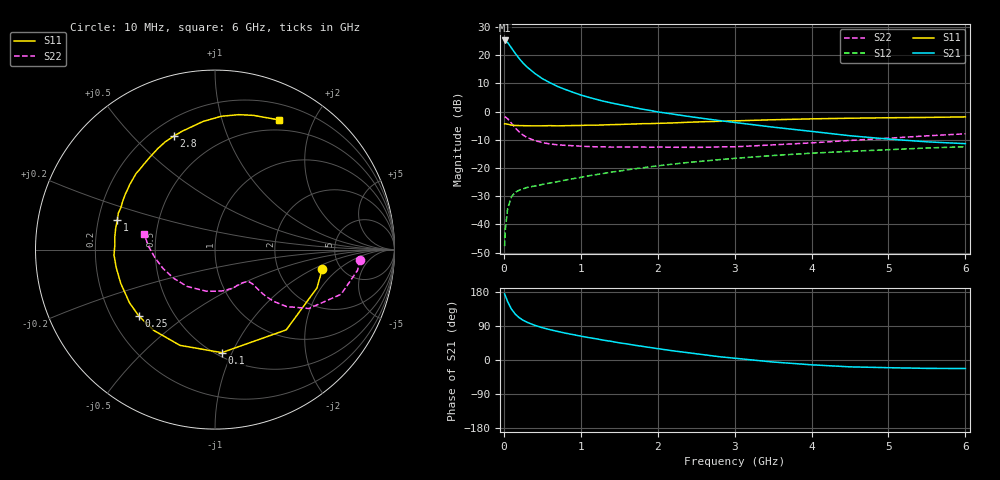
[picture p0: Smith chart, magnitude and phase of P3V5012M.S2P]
! SIEMENS Small Signal Semiconductors
! BFP181
! Si NPN RF Bipolar Junction Transistor in SOT143
! VCE = 0.5 V  IC = 12 mA
! Common Emitter S-Parameters:  March  1996
# GHz  S  MA  R  50
!  f  S11  S21  S12  S22
! GHz  MAG  ANG  MAG  ANG  MAG  ANG  MAG  ANG
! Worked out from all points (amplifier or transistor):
!   36 points, 10 MHz to 6 GHz, reference 50 ohm
!   highest |S21| = 25.2 dB at 10 MHz (marker M1)
!   |S21| within 3 dB of that: start of sweep to 108.1 MHz
!   unconditionally stable (mu >= 1): start of sweep to 15.5 MHz; 278.7 MHz to end of sweep
!   at 250 MHz: K = 0.93, MSG = 22.3 dB, |S12| = -27.4 dB
!   at 1.4 GHz: K = 2.49, MAG = 5.5 dB, |S12| = -21.5 dB
!   at 6 GHz: K = 2.44, MAG = -6.1 dB, |S12| = -12.5 dB
!   S11 on the Smith chart (normalised r, x): 10 MHz: 3.62, -1.27; 100 MHz: 0.53, -0.91; 250 MHz: 0.32, -0.34; 1 GHz: 0.28, +0.14; 2.8 GHz: 0.29, +0.66; 6 GHz: 0.37, +1.55
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0.01  0.6072 -10.5  18.29 174.5  0.0041 81.4  0.8097 -4.0
0.02  0.6069 -20.6  18.13 169.3  0.0083 75.7  0.8024 -8.3
0.05  0.598 -48.4  16.77 153.7  0.0192 67.8  0.7453 -19.5
0.1  0.5752 -86.2  13.43 134.0  0.0311 51.3  0.6175 -32.1
0.15  0.5681 -110.1  10.73 120.8  0.0372 43.0  0.5101 -38.5
0.2  0.5649 -127.1  8.731 111.6  0.0404 39.0  0.4363 -41.4
0.25  0.5629 -139.1  7.244 104.9  0.0426 36.0  0.3839 -42.6
0.3  0.561 -148.2  6.215 99.8  0.045 35.0  0.3486 -42.8
0.4  0.5579 -160.4  4.79 91.6  0.0478 35.1  0.3067 -42.5
0.5  0.5594 -169.7  3.848 85.3  0.051 35.4  0.2821 -42.5
0.6  0.5636 -176.9  3.252 80.0  0.0541 36.4  0.2666 -43.1
0.7  0.5585 177.5  2.788 75.3  0.0572 38.1  0.2574 -44.0
0.8  0.5628 172.8  2.466 70.9  0.061 38.9  0.2519 -45.1
1  0.5682 163.2  1.97 63.0  0.0682 41.0  0.2435 -48.3
1.1  0.5756 159.4  1.799 59.2  0.0726 41.5  0.2403 -50.6
1.5  0.5906 145.8  1.333 45.4  0.0882 42.4  0.235 -59.8
2.2  0.6304 125.0  0.903 24.2  0.1172 40.1  0.2331 -80.7
2.8  0.673 109.8  0.694 8.7  0.1404 35.8  0.2367 -101.6
3.5  0.7171 95.3  0.53 -5.3  0.1664 30.2  0.2571 -126.8
4.5  0.7634 80.0  0.373 -18.1  0.1974 20.7  0.3078 -159.8
5.5  0.7888 68.7  0.291 -22.1  0.2263 12.1  0.3718 177.0
6  0.8062 63.7  0.27 -22.5  0.238 7.2  0.4039 167.6
